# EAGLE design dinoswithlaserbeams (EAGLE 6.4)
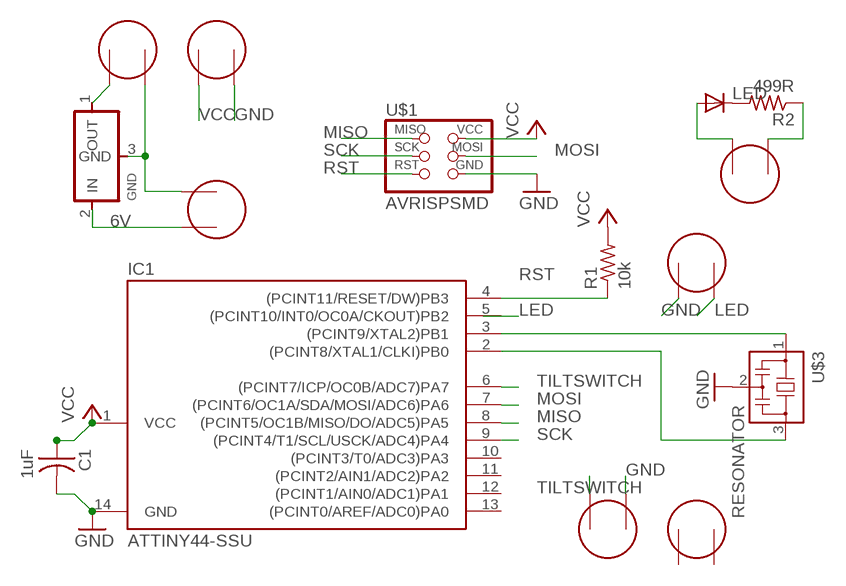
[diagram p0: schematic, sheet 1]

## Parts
C1  1uF  CAP-US1206  [C1206]
GND  REGULATORSOT23  [SOT23]
IC1  ATTINY44-SSU  [SOIC14]
LED  DIODESOD123  [SOD123]
R1  10k  RES-US1206  [R1206]
R2  499R  RES-US1206  [R1206]
U$1  AVRISPSMD  [2X03SMD]
U$2  ELECTRET  [ELECTRET_2742PBJ-A]
U$3  RESONATOR  [EFOBM]
U$4  ELECTRET  [ELECTRET_2742PBJ-A]
U$5  ELECTRET  [ELECTRET_2742PBJ-A]
U$6  ELECTRET  [ELECTRET_2742PBJ-A]
U$7  ELECTRET  [ELECTRET_2742PBJ-A]
U$8  ELECTRET  [ELECTRET_2742PBJ-A]
U$9  ELECTRET  [ELECTRET_2742PBJ-A]

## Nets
6V: GND.2(IN) U$9.P$2
GND: C1.2 IC1.14(GND) U$1.6(GND) U$3.2 U$5.P$1 U$6.P$2 U$7.P$1
LED: U$5.P$2
MISO: IC1.8((PCINT5/OC1B/MISO/DO/ADC5)PA5) U$1.1(MISO)
MOSI: IC1.7((PCINT6/OC1A/SDA/MOSI/ADC6)PA6) U$1.4(MOSI)
N$1: LED.CATHODE(C) R2.2
N$3: LED.ANODE(A) U$2.P$2
N$4: R2.1 U$2.P$1
N$5: GND.3(GND) U$8.P$2 U$9.P$1
N$6: GND.1(OUT) U$8.P$1
N$10: IC1.2((PCINT8/XTAL1/CLKI)PB0) U$3.3
N$12: IC1.3((PCINT9/XTAL2)PB1) U$3.1
RST: IC1.4((PCINT11/RESET/DW)PB3) R1.1 U$1.5(RST)
SCK: IC1.9((PCINT4/T1/SCL/USCK/ADC4)PA4) U$1.3(SCK)
TILTSWITCH: IC1.6((PCINT7/ICP/OC0B/ADC7)PA7) U$7.P$2
VCC: C1.1 IC1.1(VCC) R1.2 U$1.2(VCC) U$6.P$1
Unconnected: IC1.5((PCINT10/INT0/OC0A/CKOUT)PB2) IC1.10((PCINT3/T0/ADC3)PA3) IC1.11((PCINT2/AIN1/ADC2)PA2) IC1.12((PCINT1/AIN0/ADC1)PA1) IC1.13((PCINT0/AREF/ADC0)PA0) U$4.P$1 U$4.P$2

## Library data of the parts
C1 = fab:CAP-US
GND = fab:REGULATOR
IC1 = fab:ATTINY44
LED = fab:DIODE: DIODE
R1 R2 = fab:RES-US: Resistor (US Symbol)
U$1 = fab:AVRISP
U$2 U$4-U$9 = fab:ELECTRET
U$3 = fab:RESONATOR

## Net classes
0 default: clearance 0.355 mm

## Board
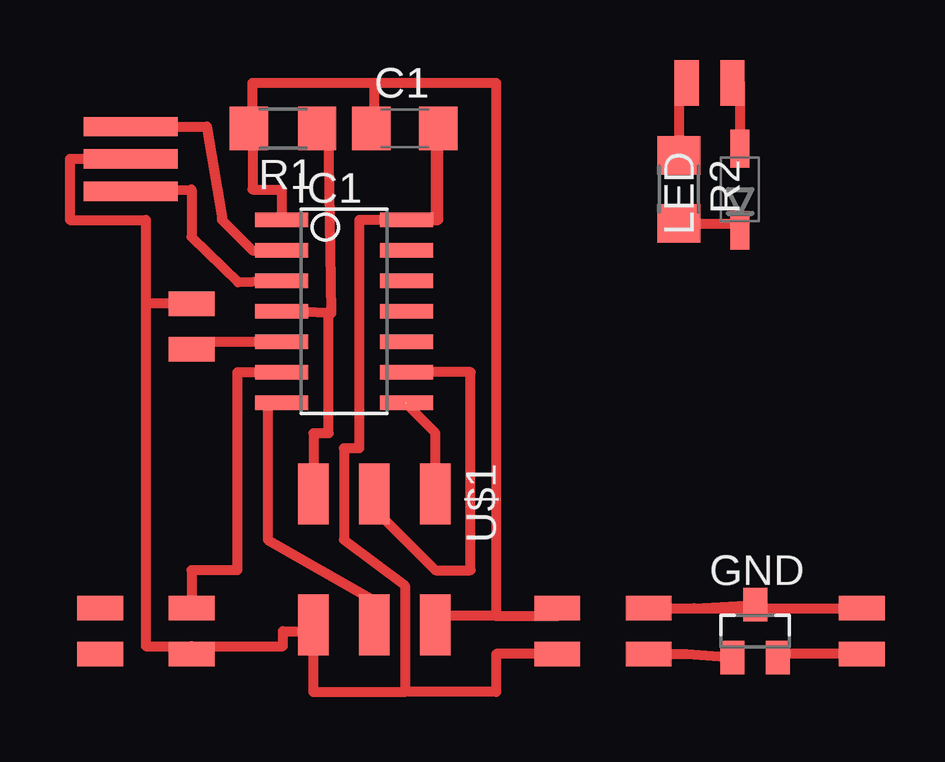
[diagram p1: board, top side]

No outline drawn. Coordinates in mm, seen from the top.
Copper layers (1*16): Top 0.035mm / dielectric 1.5mm / Bottom 0.035mm
Design rules "roy *": minimum track width 10mil, minimum drill 24mil, track to track 0.25mm, track to pad 0.25mm, pad to pad 0.25mm, via to via 0.25mm, smd to smd 0.15mm, copper to edge 40mil, drill to drill 8mil, minimum pad ring 10mil, minimum via ring 8mil, stop-mask expansion 0mil, vias tented up to drill 0mil, thermal gap 10mil

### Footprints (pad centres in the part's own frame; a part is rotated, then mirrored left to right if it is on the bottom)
C1206 = smd 1.6 x 1.8: 1 -1.4,0; 2 1.4,0
SOT23 = smd 1 x 1.4: 1 -0.95,-1.1; 2 0.95,-1.1; 3 0,1.1
SOIC14 = smd 0.61 x 2.21: 1 -3.81,-2.603; 2 -2.54,-2.603; 3 -1.27,-2.603; 4 0,-2.603; 5 1.27,-2.603; 6 2.54,-2.603; 7 3.81,-2.603; 8 3.81,2.603; 9 2.54,2.603; 10 1.27,2.603; 11 0,2.603; 12 -1.27,2.603; 13 -2.54,2.603; 14 -3.81,2.603
SOD123 = smd 1.6 x 0.8: ANODE 1.7,0; CATHODE -1.7,0
R1206 = smd 1.6 x 1.803: 1 -1.422,0; 2 1.422,0
2X03SMD = smd 2.54 x 1.27: 1 -2.54,2.54; 2 2.92,2.54; 3 -2.54,0; 4 2.92,0; 5 -2.54,-2.54; 6 2.92,-2.54
ELECTRET_2742PBJ-A = smd 1.016 x 1.905: P$1 -0.953,0; P$2 0.953,0
EFOBM = smd 0.8 x 3.9: 1 -1.35,0; 2 0,0; 3 1.35,0

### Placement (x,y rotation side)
C1  13.97,77.47 0 top
GND  28.57,56.52 0 top
IC1  11.43,69.85 270 top
LED  27.94,74.93 90 top
R1  8.89,77.47 180 top
R2  25.4,74.93 270 top
U$1  12.7,59.69 270 top
U$2  26.67,79.38 0 top
U$3  2.54,76.2 90 top
U$4  1.27,56.52 90 top
U$5  5.08,69.22 270 top
U$6  20.32,56.52 270 top
U$7  5.08,56.52 90 top
U$8  24.13,56.52 90 top
U$9  33.02,56.52 270 top

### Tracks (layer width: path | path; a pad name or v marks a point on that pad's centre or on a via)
6V
  Top 0.406: U$9.P$2 29.52,55.56 GND.2
GND
  Top 0.406: IC1.14 15.37,73.66 C1.2 | IC1.14 12.06,73.66 12.06,64.14 11.43,64.14 11.43,60.33 13.97,58.42 13.97,53.98 | 13.97,53.98 10.16,53.98 U$1.6 10.16,56.52 8.89,56.52 8.89,55.88 5.08,55.88 | 15.24,77.47 15.24,73.66 IC1.14 | U$3.2 0,76.2 0,73.66 3.17,73.66 3.17,70.17 | U$6.P$2 17.78,55.56 17.78,53.98 13.97,53.98 | 3.17,70.17 3.17,55.88 5.08,55.88 | 5.08,55.88 U$7.P$1 | U$5.P$1 3.17,70.17
MISO  (1 unrouted)
  Top 0.406: U$1.1 15.24,64.77 13.97,66.04
MOSI
  Top 0.406: IC1.7 8.26,66.04 8.26,60.33 12.7,57.78 U$1.4
N$1
  Top 0.406: R2.2 27.94,73.51 LED.CATHODE
N$2
  Top 0.406: 5.08,68.58 8.89,68.58
N$3
  Top 0.406: U$2.P$2 27.94,79.38 LED.ANODE
N$4
  Top 0.406: U$2.P$1 25.4,79.38 R2.1
N$5
  Top 0.406: GND.3 26.04,57.47 U$8.P$2 U$9.P$1
N$6
  Top 0.406: U$8.P$1 25.72,55.56 GND.1
N$10
  Top 0.406: U$3.3 5.71,77.55 6.35,73.74 6.35,73.66 7.62,72.39 IC1.2
N$12
  Top 0.406: U$3.1 5.08,74.93 5.08,72.94 7.02,71.06 IC1.3
RST
  Top 0.406: 10.91,69.78 10.79,69.85 10.79,64.77 10.16,64.77 U$1.5 | 10.91,69.78 10.79,77.47 R1.1 | IC1.4 9.64,69.85 10.91,69.78
SCK
  Top 0.406: IC1.9 16.71,67.31 16.71,59.05 15.24,59.05 12.7,61.59 U$1.3
TILTSWITCH
  Top 0.406: IC1.6 6.99,67.31 6.99,59.05 5.08,59.05 U$7.P$2
VCC
  Top 0.406: 15.62,57.15 U$1.2 15.24,57.15 17.78,57.15 | R1.2 7.62,77.47 | 7.62,77.47 7.62,79.38 12.7,79.38 | 12.7,79.38 17.78,79.38 17.78,57.15 | 7.62,77.47 7.62,74.93 8.83,74.93 IC1.1 | C1.1 12.7,77.47 12.7,79.38 | 17.78,57.15 20.32,57.15 U$6.P$1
